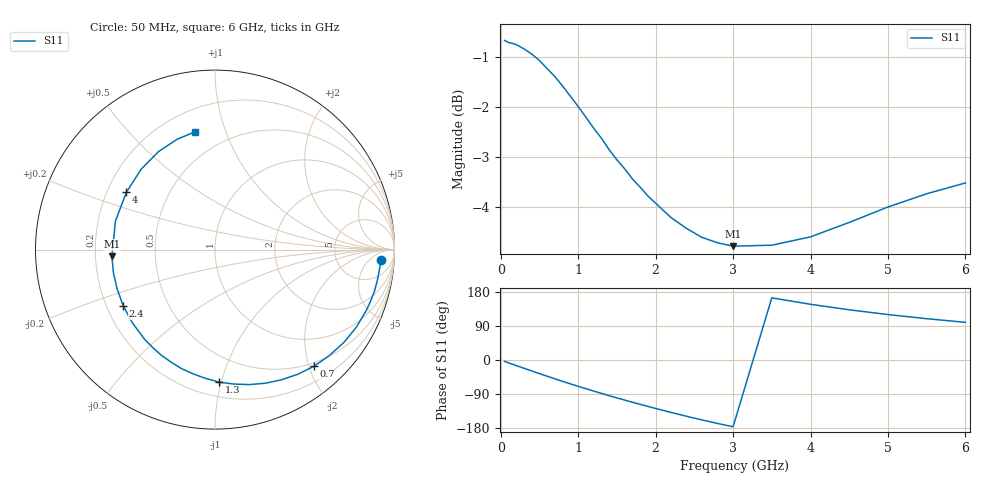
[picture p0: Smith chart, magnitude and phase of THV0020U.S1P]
! SIEMENS Discrete & RF Semiconductors
! BAS70
! Si Schottky Diode in SOT23
! IF = 0.02 mA
! S-Parameters:  February  1997
# GHz  S  MA  R  50
!  f  S11
! GHz  MAG  ANG
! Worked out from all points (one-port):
!   34 points, 50 MHz to 6 GHz, reference 50 ohm
!   lowest |S11| = -4.8 dB at 3 GHz (marker M1), VSWR 3.71, Z = 13.5 - j1.54 ohm
!   |S11| at or under -10 dB: nowhere
!   S11 on the Smith chart (normalised r, x): 50 MHz: 15, -13; 700 MHz: 0.44, -2.08; 1.3 GHz: 0.30, -0.99; 2.4 GHz: 0.27, -0.26; 4 GHz: 0.28, +0.27; 6 GHz: 0.33, +0.79
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0.05  0.9267 -3.7
0.2  0.9178 -14.7
0.3  0.9089 -21.8
0.4  0.8981 -28.9
0.5  0.8847 -35.9
0.6  0.8682 -42.9
0.7  0.8523 -49.7
0.8  0.8337 -56.4
0.9  0.8144 -63.0
1  0.7954 -69.4
1.1  0.7759 -75.8
1.2  0.7564 -82.0
1.3  0.7391 -88.1
1.4  0.7197 -94.1
1.6  0.6886 -105.8
1.8  0.66 -117.0
2  0.6359 -127.9
2.2  0.615 -138.4
2.4  0.5998 -148.5
2.6  0.5875 -158.2
2.8  0.5802 -167.4
3  0.5757 -176.2
3.5  0.577 164.0
4  0.5883 147.0
4.5  0.6082 132.5
5  0.6304 119.9
5.5  0.65 109.0
6  0.6664 99.4
